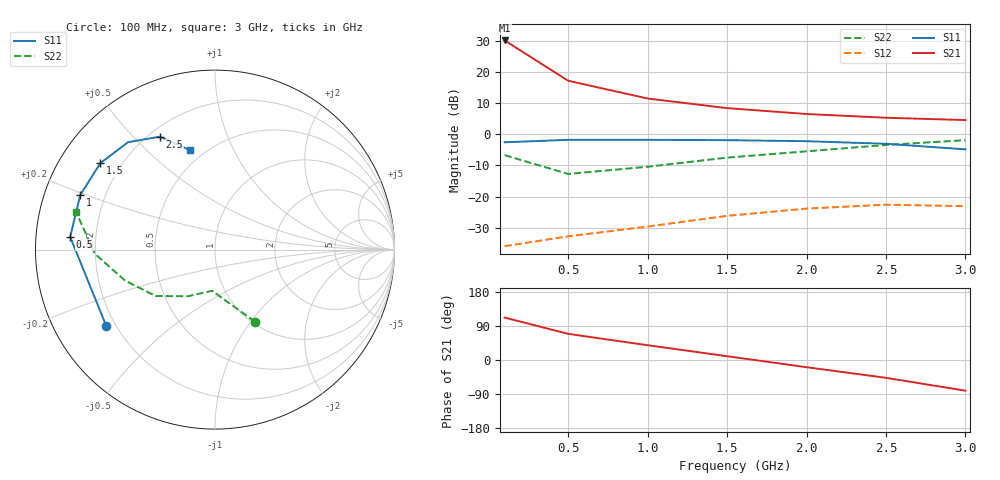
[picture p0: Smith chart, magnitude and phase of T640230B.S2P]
!AT-64023
!S-PARAMETERS at Vce=10V  Ic=150mA.  LAST UPDATED 06-28-94
# ghz s ma r 50
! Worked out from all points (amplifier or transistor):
!   7 points, 100 MHz to 3 GHz, reference 50 ohm
!   highest |S21| = 30.0 dB at 100 MHz (marker M1)
!   |S21| within 3 dB of that: start of sweep to 192.9 MHz
!   unconditionally stable (mu >= 1): 714.3 MHz to 1.485 GHz
!   at 500 MHz: K = 0.90, MSG = 24.9 dB, |S12| = -32.8 dB
!   at 1.5 GHz: K = 0.99, MSG = 17.3 dB, |S12| = -26.2 dB
!   at 3 GHz: K = 0.64, MSG = 13.8 dB, |S12| = -23.1 dB
!   S11 on the Smith chart (normalised r, x): 100 MHz: 0.16, -0.31; 500 MHz: 0.11, +0.04; 1 GHz: 0.11, +0.19; 1.5 GHz: 0.12, +0.33; 2.5 GHz: 0.24, +0.60; 3 GHz: 0.42, +0.69
0.1  0.74 -145.0  31.7 112.0  0.016 38.0  0.46 -61.0
0.5  0.81 175.0  7.17 69.0  0.023 36.0  0.23 -94.0
1  0.81 158.0  3.72 39.0  0.033 42.0  0.3 -120.0
1.5  0.8 143.0  2.61 10.0  0.049 38.0  0.42 -142.0
2  0.77 129.0  2.1 -19.0  0.064 28.0  0.53 -161.0
2.5  0.7 116.0  1.83 -47.0  0.074 12.0  0.67 -178.0
3  0.57 104.0  1.68 -81.0  0.07 -10.0  0.8 165.0
